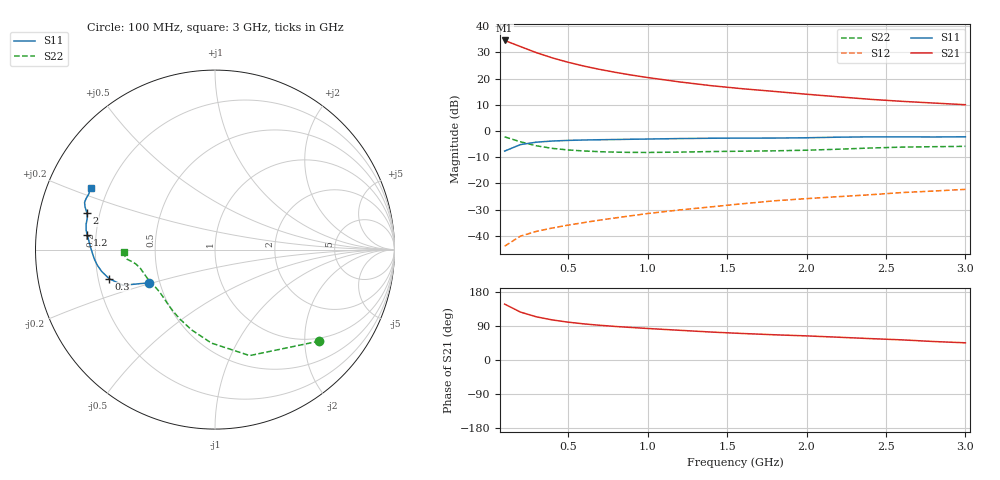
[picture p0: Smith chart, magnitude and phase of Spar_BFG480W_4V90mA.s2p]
! Filename: 490BFG480.001
! Title: BFG480W
! Bias: Vce=4V; Ic=90mA
! Company: NXP Semiconductors NL
! User: Quality&Reliability T&D
! Measure time: 10 Nov 1999 / 12:03:47
#  MHz  S  MA  R 50
! Freq  S11  S21  S12  S22  :
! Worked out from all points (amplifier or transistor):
!   20 points, 100 MHz to 3 GHz, reference 50 ohm
!   highest |S21| = 34.6 dB at 100 MHz (marker M1)
!   |S21| within 3 dB of that: start of sweep to 228.4 MHz
!   unconditionally stable (mu >= 1): 758.2 MHz to end of sweep
!   at 400 MHz: K = 0.79, MSG = 32.5 dB, |S12| = -37.1 dB
!   at 1.2 GHz: K = 1.07, MAG = 22.8 dB, |S12| = -30.2 dB
!   at 3 GHz: K = 1.04, MAG = 14.9 dB, |S12| = -22.3 dB
!   S11 on the Smith chart (normalised r, x): 100 MHz: 0.43, -0.19; 300 MHz: 0.24, -0.13; 1.2 GHz: 0.17, +0.05; 2 GHz: 0.15, +0.14; 3 GHz: 0.13, +0.23
100  0.4131 -153.4  53.56 147.5  0.006314 69.2  0.7735 -41.2
200  0.5501 -158.8  40.91 126.4  0.009832 59.9  0.6212 -71.9
300  0.612 -164.7  31.32 113.9  0.01209 58.8  0.5212 -92.2
400  0.6431 -169.1  24.9 105.8  0.01402 59.9  0.4658 -106.3
500  0.6612 -172.4  20.51 99.8  0.01596 61.9  0.4341 -116.6
600  0.6727 -175.1  17.32 95.3  0.01783 64.0  0.415 -124.3
700  0.6808 -177.5  14.97 91.6  0.01988 66.2  0.4023 -130.3
800  0.6875 -179.6  13.14 88.4  0.02194 67.9  0.3942 -135.3
900  0.6955 178.4  11.67 85.7  0.02413 69.7  0.3899 -139.6
1000  0.702 176.7  10.49 83.2  0.02651 70.9  0.3889 -143.5
1200  0.7164 173.6  8.662 78.4  0.03103 72.7  0.3951 -149.8
1400  0.7267 171.2  7.334 73.7  0.03554 73.7  0.4048 -154.4
1600  0.7317 168.9  6.398 69.9  0.04087 74.5  0.4109 -158.0
1800  0.7327 166.3  5.687 66.5  0.04647 75.2  0.418 -161.7
2000  0.7422 164.0  5.034 63.6  0.05108 75.8  0.4294 -166.1
2200  0.7615 161.9  4.493 60.1  0.05567 75.8  0.4487 -169.8
2400  0.7726 160.2  4.03 56.5  0.06054 75.3  0.473 -172.2
2600  0.7726 158.5  3.685 53.2  0.06664 74.7  0.4921 -173.7
2800  0.7684 156.2  3.417 48.8  0.07134 73.4  0.5013 -175.5
3000  0.7746 153.6  3.173 45.4  0.07674 72.5  0.5088 -178.4
